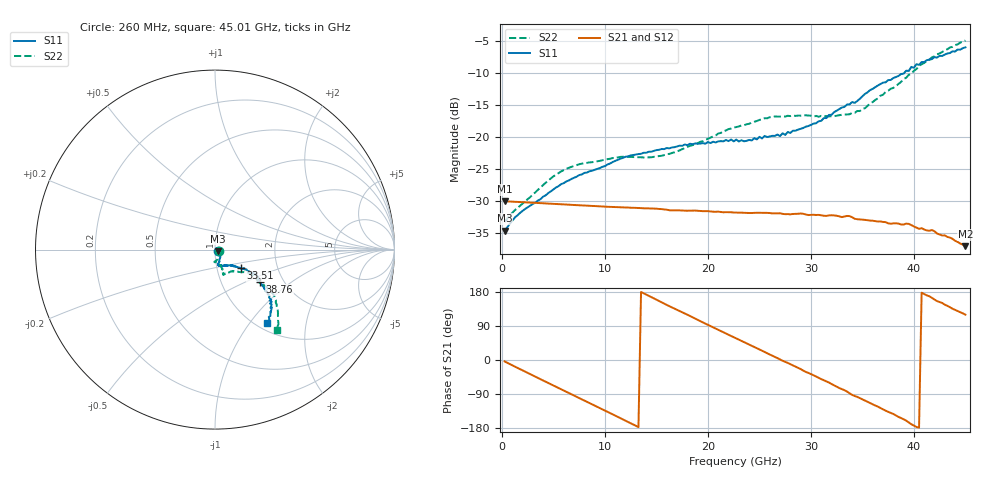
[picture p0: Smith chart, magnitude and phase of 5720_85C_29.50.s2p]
! Device:  ADRF5720
! Description: 0.5dB LSB GaAs MMIC 6-bit Digital Attenuator
! Frequency:  0.000009 -  40 GHz
! Ports:
!	RF1	= Port 1
!	RF2	= Port 2
! Vdd:  3.3 Volt
! Vss:  -3.3 Volt
! Control:  0/3.3 Volt
! State:  29.50 dB attenuation
! Data:  The device was measured using G-S-G Probes on a matrix board.
!  Data was collected using an calibrated 4 port network analyzer.
!  The reference plane for this measurement is at the launchers.
! Note:  Analog Devices supplies this data as a sample of measured data
!  for this product.  Your particular data for this product may vary.
!  Data was taken at 85 degrees C.
!  Analog Devices reserves the right to change this data at anytime.
# GHZ S DB R 45.0
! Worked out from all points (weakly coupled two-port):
!   180 points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, 260 MHz to 45.01 GHz, reference 45 ohm
!   highest |S21| = -30.01 dB at 260 MHz (marker M1); lowest = -37.0 dB at 45.01 GHz (marker M2)
!   lowest |S11| = -34.6 dB at 260 MHz (marker M3), VSWR 1.04, Z = 46.6 - j0.718 ohm
!   |S11| at or under -10 dB: start of sweep to 39.07 GHz
!   |S22| runs from -33.3 to -4.9 dB; largest |S21 - S12| = 0.00022
!   S11 on the Smith chart (normalised r, x): 260 MHz: 1.03, -0.02; 33.51 GHz: 1.31, -0.28; 38.76 GHz: 1.52, -0.61; 45.01 GHz: 1.12, -1.22
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0.26  -34.57 -24.4  -30.01 -3.7  -30.01 -3.7  -33.26 -22.7
1.76  -31.82 -4.4  -30.14 -24.2  -30.12 -24.1  -30.71 -21.4
5.01  -28.14 -40.3  -30.41 -67.4  -30.40 -67.3  -26.12 -68.4
7.76  -25.83 -54.7  -30.65 -103.8  -30.64 -103.7  -24.15 -83.4
12.01  -23.06 -69.8  -30.98 -160.2  -30.96 -160.0  -23.06 -91.8
15.26  -21.99 -76.1  -31.21 155.6  -31.19 155.7  -22.96 -84.9
17.26  -21.34 -78.9  -31.43 129.4  -31.42 129.5  -22.08 -78.7
22.76  -20.39 -72.4  -31.77 56.8  -31.76 57.0  -18.44 -69.6
23.51  -20.66 -71.8  -31.81 47.1  -31.80 47.3  -18.16 -69.4
25.51  -19.82 -64.5  -31.81 21.3  -31.80 21.6  -17.06 -71.6
27.01  -19.85 -59.2  -31.88 1.4  -31.87 1.8  -16.81 -70.7
30.26  -17.90 -45.4  -32.11 -40.3  -32.09 -40.1  -16.81 -70.1
33.51  -14.93 -35.4  -32.30 -83.3  -32.30 -83.0  -16.47 -55.6
34.26  -14.67 -36.5  -32.74 -95.1  -32.73 -94.8  -16.23 -50.5
35.26  -13.27 -33.4  -32.91 -106.9  -32.89 -106.6  -15.50 -45.9
37.76  -11.10 -32.1  -33.51 -139.7  -33.47 -139.4  -12.47 -34.5
38.76  -10.18 -35.7  -33.62 -153.2  -33.57 -153.0  -11.41 -34.6
39.51  -9.69 -36.9  -33.54 -164.9  -33.50 -164.3  -10.30 -36.3
40.26  -8.64 -39.0  -34.12 -176.7  -34.07 -176.2  -9.40 -36.0
41.76  -7.84 -41.6  -34.50 163.8  -34.47 164.1  -7.57 -37.9
43.51  -6.90 -45.5  -35.67 139.3  -35.63 139.7  -6.03 -45.3
45.01  -6.01 -54.3  -37.01 119.7  -36.96 120.0  -4.94 -52.2
